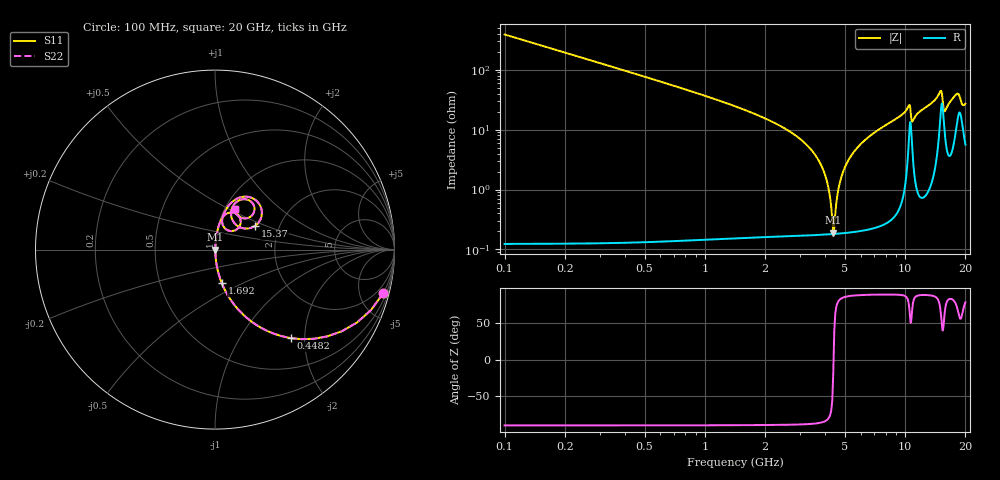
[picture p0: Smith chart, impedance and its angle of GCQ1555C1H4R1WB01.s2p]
!Murata Part Number: GCQ1555C1H4R1WB01
!These Parameters are Measured in Series Mode Connection
!Data Generated on Mar 13, 2026
!  o--ll--o
!Port1  Port2
!  o------o
!Operation Temp=25[degC], DC Bias Voltage=0[V]
!Freq. Start=100[MHz] Stop=20[GHz] 401[Steps]
# Hz S RI R 50
!Freq.(Hz) S11(Real) S11(Imag) S21(Real) S21(Imag) S12(Real) S12(Imag) S22(Real) S22(Imag)
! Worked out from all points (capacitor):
!   401 points, 100 MHz to 20 GHz, reference 50 ohm
!   read as one part in series: C = 4.1 pF near 199.5 MHz
!   lowest |Z| = 190 mohm at 4.378 GHz (marker M1)
!   series resonance near 4.393 GHz, so ESL is about 320 pH
!   S11 on the Smith chart (normalised r, x): 100 MHz: 1.00, -7.76; 448.2 MHz: 1.00, -1.71; 1.692 GHz: 1.00, -0.39; 15.37 GHz: 1.50, +0.42; 20 GHz: 1.11, +0.53
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1e8  0.9376 -0.2417  0.0624 0.2417  0.0624 0.2417  0.9376 -0.2417
4.4825e8  0.4235 -0.4934  0.5765 0.4934  0.5765 0.4934  0.4235 -0.4934
8.96e8  0.1479 -0.3533  0.8521 0.3533  0.8521 0.3533  0.1479 -0.3533
1.692e9  0.0382 -0.1878  0.9618 0.1878  0.9618 0.1878  0.0382 -0.1878
3.43325e9  0.00367 -0.044  0.9963 0.044  0.9963 0.044  0.00367 -0.044
4.03025e9  0.00201 -0.0153  0.998 0.0153  0.998 0.0153  0.00201 -0.0153
4.3785e9  0.00181 -0.000569  0.9982 0.000569  0.9982 0.000569  0.00181 -0.000569
4.478e9  0.00183 0.00343  0.9982 -0.00343  0.9982 -0.00343  0.00183 0.00343
4.72675e9  0.00202 0.0131  0.998 -0.0131  0.998 -0.0131  0.00202 0.0131
5.075e9  0.00256 0.0259  0.9974 -0.0259  0.9974 -0.0259  0.00256 0.0259
6.7665e9  0.00874 0.0805  0.9913 -0.0805  0.9913 -0.0805  0.00874 0.0805
1.005e10  0.051 0.1898  0.949 -0.1898  0.949 -0.1898  0.051 0.1898
1.049775e10  0.1268 0.194  0.8732 -0.194  0.8732 -0.194  0.1268 0.194
1.0846e10  0.0616 0.1129  0.9384 -0.1129  0.9384 -0.1129  0.0616 0.1129
1.338325e10  0.0764 0.2453  0.9236 -0.2453  0.9236 -0.2453  0.0764 0.2453
1.497525e10  0.2268 0.2754  0.7732 -0.2754  0.7732 -0.2754  0.2268 0.2754
1.537325e10  0.2215 0.1307  0.7785 -0.1307  0.7785 -0.1307  0.2215 0.1307
1.57215e10  0.1132 0.1424  0.8868 -0.1424  0.8868 -0.1424  0.1132 0.1424
1.67165e10  0.1031 0.2469  0.8969 -0.2469  0.8969 -0.2469  0.1031 0.2469
1.85075e10  0.2199 0.2276  0.7801 -0.2276  0.7801 -0.2276  0.2199 0.2276
1.93035e10  0.145 0.178  0.855 -0.178  0.855 -0.178  0.145 0.178
2e10  0.1096 0.2239  0.8904 -0.2239  0.8904 -0.2239  0.1096 0.2239
